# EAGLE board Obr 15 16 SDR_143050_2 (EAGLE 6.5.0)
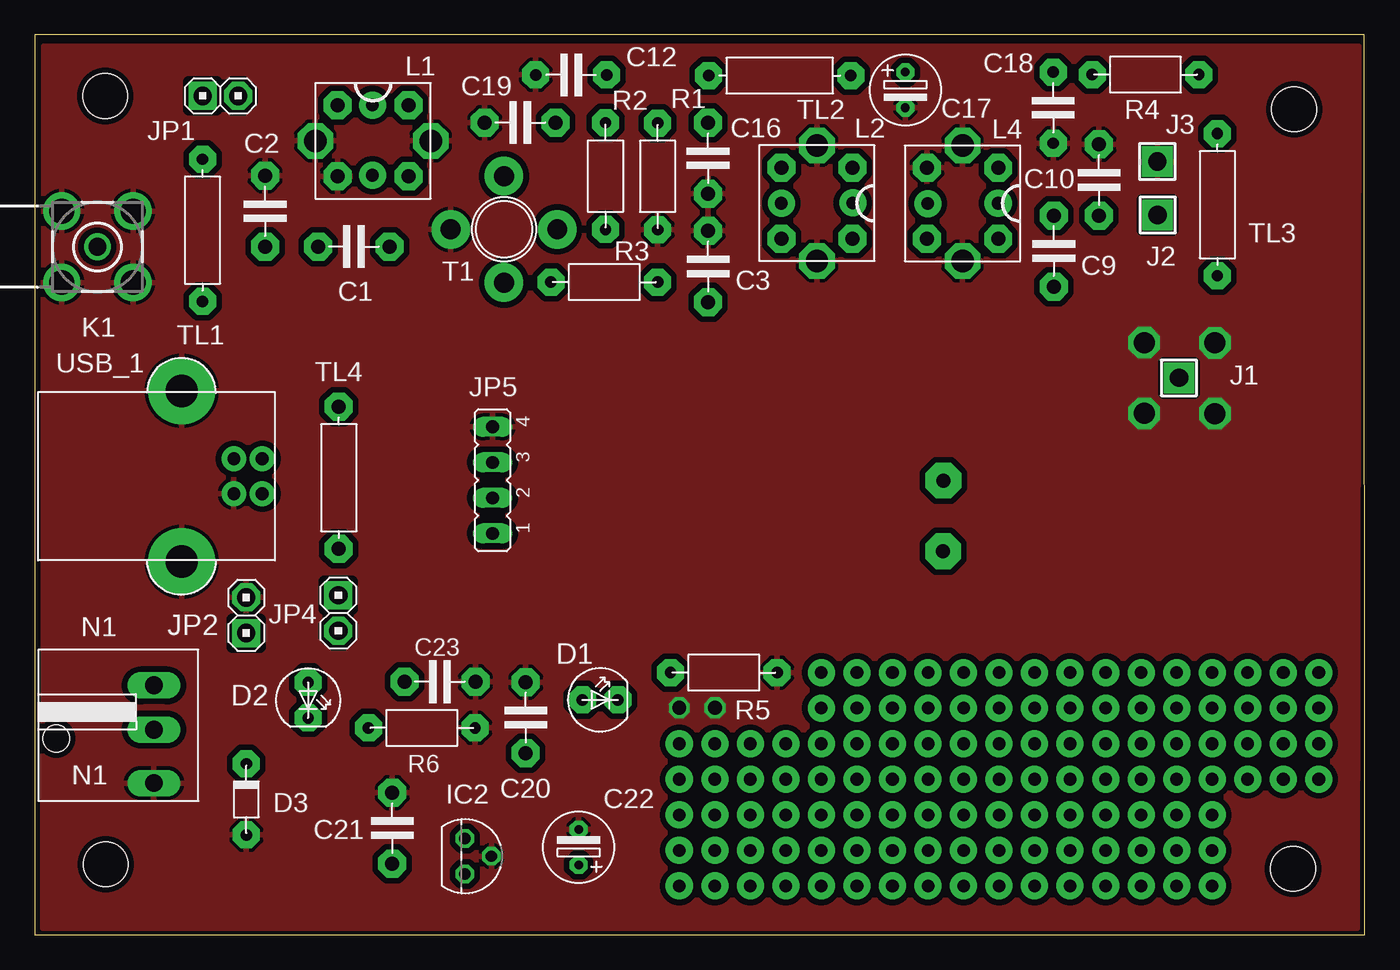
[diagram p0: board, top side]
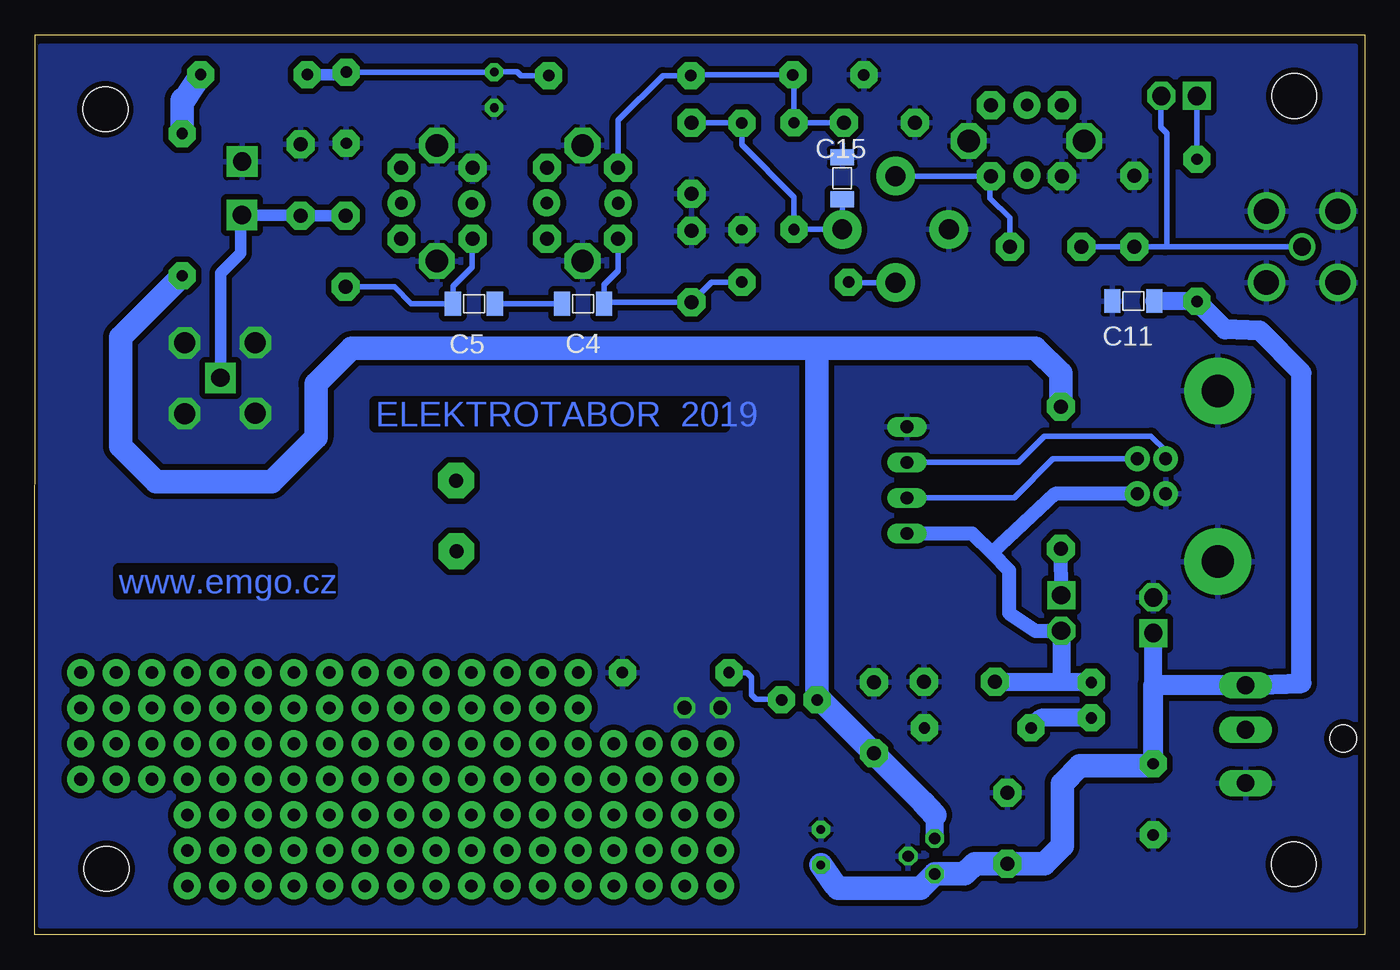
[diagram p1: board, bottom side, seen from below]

Size 95.05 x 64.29 mm. Coordinates in mm from the lower left corner, seen from the top.
Outline: 0,0 95.05,0 95.02,64.29 0,64.29 0,0
Copper layers (1*16): Top 0.035mm / dielectric 1.5mm / Bottom 0.035mm
Design rules "default *": minimum track width 10mil, minimum drill 24mil, track to track 8mil, track to pad 8mil, pad to pad 8mil, via to via 8mil, smd to smd 8mil, copper to edge 0mil, drill to drill 8mil, minimum pad ring 10mil, minimum via ring 8mil, stop-mask expansion 4mil, vias tented up to drill 0mil, thermal gap 10mil
Holes 3.2 mm at 5.05,5.02 90.01,59 89.94,4.72 5.02,59.94

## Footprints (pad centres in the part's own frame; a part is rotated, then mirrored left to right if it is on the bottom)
C-5 = drill 1 pad 2 octagon: 1 -2.54,0; 2 2.54,0
SMD-1206 = smd 1.15 x 1.7: 1 -1.5,0; 2 1.5,0
C-5@2 = drill 0.813 pad 1.93 octagon: 1 -2.54,0; 2 2.54,0
ES-2,5L = drill 0.61 pad 1.27 octagon: 1 0,0; 2 2.54,0
LED = drill 0.813 pad 1.93 octagon: A 0,0; K 2.54,0
D-5 = drill 0.813 pad 1.93 octagon: 1 -2.54,0; 2 2.54,0
TO92 = drill 0.813 octagon: 1 -1.27,0; 2 0,1.905; 3 1.27,0
PAD-01 = drill 1.3 pad 2.184 square: 1 0,0
PINH-2 = drill 1.3 pad 2 square: 1 0,0 | drill 1.3 pad 2 octagon: 2 2.54,0
JP4 = drill 0.914 long: 1 -3.81,0; 2 -1.27,0; 3 1.27,0; 4 3.81,0
BU-SMA-H = drill 1.27: 1 0,0 | drill 1.778: 2 -2.55,2.55; 3 2.55,2.55; 4 2.55,-2.55; 5 -2.55,-2.55
L-VF50 = drill 1 pad 2 octagon: 1 -2.54,-2.54; 2 2.54,-2.54; 3 2.54,2.54; 4 -2.54,2.54 | drill 1.6 pad 2.54 octagon: 5 -4.128,0; 6 4.128,0
NAPVIDL = drill 1.27 pad 1.905 long: 1 3.175,0; 2 -3.81,0; 3 0,0 | hole 1.93: -0.635,6.985
R-7,5 = drill 0.813 pad 1.93 octagon: 1 -3.81,0; 2 3.81,0
BF982 = drill 1.422 pad 2.75: 1 -3.81,0; 2 0,3.81; 3 3.81,0; 4 0,-3.81
L-10@2 = drill 0.813 pad 1.93 octagon: 1 -5.08,0; 2 5.08,0
L-10 = drill 1 pad 2 octagon: 1 -5.08,0; 2 5.08,0
USB1X90B = drill 0.92 pad 1.778: 1 -1.016,1.245; 2 -1.016,-1.245; 3 1.016,-1.245; 4 1.016,1.245 | drill 2.3 pad 4.778: P$3 4.75,-6.096; P$4 4.75,6.096

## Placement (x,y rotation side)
C1  5.6pF  [C-5]  22.8,49.17 0 top
C2  33pF  [C-5]  16.45,51.7 270 top
C3  8.2pF  [C-5]  48.12,47.75 270 top
C4  1pF  [SMD-1206]  55.87,45.09 0 bottom
C5  1pF  [SMD-1206]  63.67,45.09 0 bottom
C9  4.7pF  [C-5]  72.84,48.85 270 top
C10  33pF  [C-5]  76.07,53.93 270 top
C11  100nF  [SMD-1206]  16.53,45.28 180 bottom
C12  100nF  [C-5@2]  38.33,61.44 0 top
C15  1nF  [SMD-1206]  37.33,54.04 90 bottom
C16  100nF  [C-5]  48.12,55.48 270 top
C17  47uF  [ES-2,5L]  62.23,61.63 270 top
C18  100nF  [C-5@2]  72.79,59.1 90 top
C19  1nF  [C-5]  34.69,58.03 180 top
C20  100nF  [C-5]  35.08,15.51 270 top
C21  100nF  [C-5]  25.55,7.61 270 top
C22  47uF  [ES-2,5L]  38.86,4.98 90 top
C23  100nF  [C-5]  28.95,18.08 0 top
D1  RED/5mA  [LED]  39.14,16.78 0 top
D2  RED/5mA  [LED]  19.53,18.03 270 top
D3  protect  [D-5]  15.11,9.67 90 top
IC2  78L08Z  [TO92]  30.73,5.61 270 top
J1  [PAD-01]  81.78,39.8 90 top
J2  [PAD-01]  80.26,51.43 0 top
J3  [PAD-01]  80.23,55.25 0 top
JP1  [PINH-2]  11.98,59.94 0 top
JP2  UCC-GND  [PINH-2]  15.11,21.56 90 top
JP4  USB-GND  [PINH-2]  21.69,24.25 270 top
JP5  [JP4]  32.71,32.48 90 top
K1  [BU-SMA-H]  4.47,49.16 180 top
L1  [L-VF50]  24.17,56.73 0 top
L2  [L-VF50]  55.9,52.27 270 top
L4  [L-VF50]  66.31,52.26 270 top
N1  12V-DC  [NAPVIDL]  8.5,14.65 90 top
R1  100K  [R-7,5]  44.51,54.18 270 top
R2  100K  [R-7,5]  40.79,54.21 90 top
R3  47R  [R-7,5]  40.7,46.63 180 top
R4  2R2  [R-7,5]  79.39,61.46 180 top
R5  1K  [R-7,5]  49.24,18.73 180 top
R6  1K  [R-7,5]  27.66,14.78 180 top
T1  BF982A  [BF982]  33.53,50.4 0 top
TL1  10uH  [L-10@2]  11.98,50.34 270 top
TL2  TLUM  [L-10@2]  53.24,61.39 0 top
TL3  TLUM  [L-10@2]  84.53,52.17 270 top
TL4  10uH  [L-10]  21.72,32.65 270 top
USB_1  [USB1X90B]  15.24,32.76 180 top

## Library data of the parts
C1-C5 C9-C12 C15-C23 D1-D3 J1-J3 JP1 JP2 JP4 L1 L2 L4 N1 R1-R6 TL1-TL4 = M
IC2 = linear
JP5 = jumper
K1 = con-coax; OC_FARNELL: unknown; OC_NEWARK: unknown
T1 = transistor-fet
USB_1 = EMGO_BNC

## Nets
+12V: C11.1 C21.2 C22.1 D3.2 IC2.3 JP2.1 N1.1 TL1.2
+12V1: C23.1 D2.A JP4.2 JP5.1 USB_1.1
+12V2: C20.2 D1.A IC2.1 TL3.2 TL4.1
GND: C2.1 C3.1 C10.1 C11.2 C12.1 C15.2 C16.2 C17.2 C18.1 C19.2 C20.1 C21.1 C22.2 C23.2 D3.1 IC2.2 J3.1 JP2.2 JP5.4 K1.2 K1.3 K1.4 K1.5 L1.1 L1.5 L1.6 L2.5 L2.6 L4.1 L4.5 L4.6 N1.2 R1.2 R5.1 R6.1 T1.1 USB_1.4 USB_1.P$3 USB_1.P$4
N$1: R4.1 TL3.1
N$2: R3.2 T1.4
N$8: D2.K R6.2
N$10: JP5.2 USB_1.2
N$13: C17.1 C18.2 R4.2 TL2.2
N$14: JP5.3 USB_1.3
N$16: C4.1 C5.2
N$29: C5.1 C9.2 L4.2
N$30: C9.1 C10.2 J1.1 J2.1
N$34: JP1.1 TL1.1
N$36: C3.2 C4.2 L2.2 R3.1
N$38: C12.2 C19.1 L2.1 R2.2 TL2.1
N$44: C1.2 L1.2 T1.2
N$45: C1.1 C2.2 JP1.2 K1.1
N$50: C15.1 C16.1 R1.1 R2.1 T1.3
N$85: D1.K R5.2
N$146: JP4.1 TL4.2

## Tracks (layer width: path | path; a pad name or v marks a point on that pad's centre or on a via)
+12V
  Bottom 0.406: 15.03,45.26 C11.1
  Bottom 1.27: TL1.2 15.01,45.26 C11.1 | 15.11,17.82 JP2.1
  Bottom 1.422: TL1.2 9.98,43.25 7.49,43.17 4.52,40.15 4.52,17.98 N1.1 15.11,17.82 D3.2
  Bottom 1.676: C22.1 37.91,3.59 37.64,3.32 31.75,3.32 IC2.3 28.6,4.34 27.86,5.07 C21.2 22.88,5.07 21.61,6.34 21.61,10.79 20.34,12.06 15.26,12.06 D3.2
+12V1
  Bottom 1.016: JP5.1 28.06,28.67 26.65,27.31 | 26.65,27.31 25.42,26.03 25.42,22.98 23.52,21.71 JP4.2 | USB_1.1 22.13,31.5 26.65,27.31
  Bottom 1.27: C23.1 21.61,18.08 | 21.61,18.08 19.58,18.08 D2.A | JP4.2 21.69,18.15 21.61,18.08
+12V2
  Bottom 1.27: IC2.1 30.73,8.54
  Bottom 1.676: TL4.1 21.72,40.11 23.52,41.9 39.39,41.9 | 39.39,41.9 72.41,41.9 74.95,39.36 74.95,35.55 78.13,32.38 86.38,32.38 88.92,34.92 88.92,42.69 TL3.2 | 39.39,41.9 39.14,41.65 D1.A 38.89,16.78 C20.2 31.6,9.49 30.73,8.54
GND  (via drill 1 pad 1.02, 1.5)
  other vias: 46.06,16.21 48.62,16.21 79.29,42.31 84.35,42.28 84.35,37.23 79.29,37.26
  pour Bottom (isolate 0.406): 0.66,0.63 0.66,63.49 94.64,63.49 94.64,0.63
  pour Top (isolate 0.406): 0.63,63.49 94.64,63.49 94.53,0.48 0.55,0.48
N$1
  Bottom 1.676: TL3.1 84.53,59.63 84.48,59.68 84.34,59.68 R4.1
N$2
  Bottom 0.406: T1.4 36.84,46.59 R3.2
N$3  (via drill 0.9 pad 1.93)
  other vias: 46.06,13.65
N$8
  Bottom 1.27: D2.K 23.13,15.49 R6.2
N$9  (via drill 0.9 pad 1.93)
  other vias: 48.6,13.65
N$10
  Bottom 0.406: USB_1.2 22.27,34 25.04,31.24 JP5.2
N$11  (via drill 0.9 pad 1.93)
  other vias: 51.14,13.65
N$12  (via drill 0.9 pad 1.93)
  other vias: 53.68,13.65
N$13
  Bottom 0.406: C18.2 C17.1 62.19,61.66 60.57,61.66 60.3,61.39 TL2.2
  Bottom 0.813: R4.2 72.96,61.46 C18.2
N$14
  Bottom 0.406: JP5.3 24.73,33.78 22.88,35.63 15.26,35.63 14.22,34.59 USB_1.3
N$15  (via drill 0.9 pad 1.93)
  other vias: 46.06,11.11
N$16
  Bottom 0.406: C4.1 C5.2
N$17  (via drill 0.9 pad 1.93)
  other vias: 48.6,11.11
N$19  (via drill 0.9 pad 1.93)
  other vias: 51.14,11.11
N$20  (via drill 0.9 pad 1.93)
  other vias: 53.68,11.11
N$21  (via drill 0.9 pad 1.93)
  other vias: 46.06,8.57
N$22  (via drill 0.9 pad 1.93)
  other vias: 48.6,8.57
N$23  (via drill 0.9 pad 1.93)
  other vias: 51.14,8.57
N$24  (via drill 0.9 pad 1.93)
  other vias: 53.68,8.57
N$25  (via drill 0.9 pad 1.93)
  other vias: 48.6,6.03
N$26  (via drill 0.9 pad 1.93)
  other vias: 53.68,6.03
N$27  (via drill 0.9 pad 1.93)
  other vias: 51.14,6.03
N$28  (via drill 0.9 pad 1.93)
  other vias: 46.06,6.03
N$29
  Bottom 0.406: L4.2 63.8,49.69 63.8,47.69 65.17,46.32 C5.1 65.19,45.1 68.14,45.1 69.35,46.31 C9.2
N$30
  Bottom 0.813: C9.1 C10.2 76.11,51.43 J2.1 80.34,51.35 80.34,48.71 81.78,47.26 J1.1
N$31  (via drill 0.9 pad 1.93)
  other vias: 46.06,3.49
N$32  (via drill 0.9 pad 1.93)
  other vias: 48.6,3.49
N$33  (via drill 0.9 pad 1.93)
  other vias: 51.14,3.49
N$34
  Bottom 0.406: TL1.1 JP1.1
N$35  (via drill 0.9 pad 1.93)
  other vias: 53.68,3.49
N$36
  Bottom 0.406: L2.2 53.36,47.44 54.37,46.43 C4.2 54.25,45.21 C3.2 46.7,46.63 R3.1
N$37  (via drill 0.9 pad 1.93)
  other vias: 56.22,3.49
N$38
  Bottom 0.406: C19.1 40.77,58.03 R2.2 40.79,61.35 C12.2 48.12,61.44 TL2.1 50.16,61.39 53.36,58.18 L2.1
N$39  (via drill 0.9 pad 1.93)
  other vias: 56.22,6.03
N$40  (via drill 0.9 pad 1.93)
  other vias: 56.22,8.57
N$41  (via drill 0.9 pad 1.93)
  other vias: 56.22,11.11
N$42  (via drill 0.9 pad 1.93)
  other vias: 56.22,13.65
N$43  (via drill 0.9 pad 1.93)
  other vias: 56.22,16.19
N$44
  Bottom 0.406: T1.2 33.53,54.19 L1.2 26.77,54.13 26.77,52.62 25.37,51.23 25.37,49.17 C1.2
N$45
  Bottom 0.406: K1.1 14.27,49.16 | 14.27,49.16 C2.2 C1.1 | 14.27,49.16 14.14,49.28 14.14,57.27 14.57,57.7 14.57,59.89 JP1.2
N$46  (via drill 0.9 pad 1.93)
  other vias: 56.22,18.73
N$47  (via drill 0.9 pad 1.93)
  other vias: 58.76,6.03
N$48  (via drill 0.9 pad 1.93)
  other vias: 58.76,16.19
N$49  (via drill 0.9 pad 1.93)
  other vias: 58.76,13.65
N$50
  Bottom 0.406: 37.33,50.41 T1.3 | T1.3 R2.1 40.79,52.7 44.52,56.43 R1.1 44.54,58.02 C16.1 | T1.3 C15.1
N$51  (via drill 0.9 pad 1.93)
  other vias: 58.76,11.11
N$52  (via drill 0.9 pad 1.93)
  other vias: 58.76,8.57
N$53  (via drill 0.9 pad 1.93)
  other vias: 58.76,3.49
N$54  (via drill 0.9 pad 1.93)
  other vias: 58.76,18.73
N$55  (via drill 0.9 pad 1.93)
  other vias: 61.3,6.03
N$56  (via drill 0.9 pad 1.93)
  other vias: 61.3,16.19
N$57  (via drill 0.9 pad 1.93)
  other vias: 61.3,13.65
N$58  (via drill 0.9 pad 1.93)
  other vias: 61.3,11.11
N$59  (via drill 0.9 pad 1.93)
  other vias: 61.3,8.57
N$60  (via drill 0.9 pad 1.93)
  other vias: 84.16,6.03
N$61  (via drill 0.9 pad 1.93)
  other vias: 61.3,3.49
N$62  (via drill 0.9 pad 1.93)
  other vias: 63.84,3.49
N$63  (via drill 0.9 pad 1.93)
  other vias: 63.84,6.03
N$64  (via drill 0.9 pad 1.93)
  other vias: 63.84,8.57
N$65  (via drill 0.9 pad 1.93)
  other vias: 63.84,11.11
N$66  (via drill 0.9 pad 1.93)
  other vias: 63.84,13.65
N$67  (via drill 0.9 pad 1.93)
  other vias: 63.84,16.19
N$68  (via drill 0.9 pad 1.93)
  other vias: 61.3,18.73
N$69  (via drill 0.9 pad 1.93)
  other vias: 63.84,18.73
N$70  (via drill 0.9 pad 1.93)
  other vias: 66.38,6.03
N$71  (via drill 0.9 pad 1.93)
  other vias: 66.38,18.73
N$72  (via drill 0.9 pad 1.93)
  other vias: 66.38,16.19
N$73  (via drill 0.9 pad 1.93)
  other vias: 66.38,13.65
N$74  (via drill 0.9 pad 1.93)
  other vias: 66.38,11.11
N$75  (via drill 0.9 pad 1.93)
  other vias: 66.38,8.57
N$76  (via drill 0.9 pad 1.93)
  other vias: 24.12,54.27
N$77  (via drill 0.9 pad 1.93)
  other vias: 24.12,59.28
N$78  (via drill 0.9 pad 1.93)
  other vias: 53.36,52.27
N$79  (via drill 0.9 pad 1.93)
  other vias: 58.47,52.29
N$80  (via drill 0.9 pad 1.93)
  other vias: 63.83,52.24
N$81  (via drill 0.9 pad 1.93)
  other vias: 68.85,52.27
N$82  (via drill 1 pad 2.54)
  other vias: 64.94,32.45
N$83  (via drill 1 pad 2.54)
  other vias: 64.92,27.4
N$84  (via drill 0.9 pad 1.93)
  other vias: 66.38,3.49
N$85
  Bottom 0.406: R5.2 44.16,18.73 43.84,18.41 43.84,17.14 43.52,16.82 41.71,16.82 D1.K
N$86  (via drill 0.9 pad 1.93)
  other vias: 68.92,3.49
N$87  (via drill 0.9 pad 1.93)
  other vias: 68.92,6.03
N$88  (via drill 0.9 pad 1.93)
  other vias: 68.92,8.57
N$89  (via drill 0.9 pad 1.93)
  other vias: 68.92,11.11
N$90  (via drill 0.9 pad 1.93)
  other vias: 68.92,13.65
N$91  (via drill 0.9 pad 1.93)
  other vias: 68.92,16.19
N$92  (via drill 0.9 pad 1.93)
  other vias: 68.92,18.73
N$93  (via drill 0.9 pad 1.93)
  other vias: 71.46,6.03
N$94  (via drill 0.9 pad 1.93)
  other vias: 71.46,18.73
N$95  (via drill 0.9 pad 1.93)
  other vias: 71.46,16.19
N$96  (via drill 0.9 pad 1.93)
  other vias: 71.46,13.65
N$97  (via drill 0.9 pad 1.93)
  other vias: 71.46,11.11
N$98  (via drill 0.9 pad 1.93)
  other vias: 71.46,8.57
N$99  (via drill 0.9 pad 1.93)
  other vias: 71.46,3.49
N$100  (via drill 0.9 pad 1.93)
  other vias: 74,3.49
N$101  (via drill 0.9 pad 1.93)
  other vias: 74,6.03
N$102  (via drill 0.9 pad 1.93)
  other vias: 74,8.57
N$103  (via drill 0.9 pad 1.93)
  other vias: 74,11.11
N$104  (via drill 0.9 pad 1.93)
  other vias: 74,13.65
N$105  (via drill 0.9 pad 1.93)
  other vias: 74,16.19
N$106  (via drill 0.9 pad 1.93)
  other vias: 74,18.73
N$107  (via drill 0.9 pad 1.93)
  other vias: 76.54,6.03
N$108  (via drill 0.9 pad 1.93)
  other vias: 76.54,16.19
N$109  (via drill 0.9 pad 1.93)
  other vias: 76.54,13.65
N$110  (via drill 0.9 pad 1.93)
  other vias: 76.54,11.11
N$111  (via drill 0.9 pad 1.93)
  other vias: 76.54,8.57
N$112  (via drill 0.9 pad 1.93)
  other vias: 76.54,3.49
N$113  (via drill 0.9 pad 1.93)
  other vias: 79.08,3.49
N$114  (via drill 0.9 pad 1.93)
  other vias: 79.08,6.03
N$115  (via drill 0.9 pad 1.93)
  other vias: 79.08,8.57
N$116  (via drill 0.9 pad 1.93)
  other vias: 79.08,11.11
N$117  (via drill 0.9 pad 1.93)
  other vias: 79.08,13.65
N$118  (via drill 0.9 pad 1.93)
  other vias: 79.08,16.19
N$119  (via drill 0.9 pad 1.93)
  other vias: 76.54,18.73
N$120  (via drill 0.9 pad 1.93)
  other vias: 79.08,18.73
N$121  (via drill 0.9 pad 1.93)
  other vias: 81.62,18.73
N$122  (via drill 0.9 pad 1.93)
  other vias: 84.16,18.73
N$123  (via drill 0.9 pad 1.93)
  other vias: 86.7,18.73
N$124  (via drill 0.9 pad 1.93)
  other vias: 89.24,18.73
N$125  (via drill 0.9 pad 1.93)
  other vias: 91.78,18.73
N$126  (via drill 0.9 pad 1.93)
  other vias: 86.7,16.19
N$127  (via drill 0.9 pad 1.93)
  other vias: 91.78,16.19
N$128  (via drill 0.9 pad 1.93)
  other vias: 89.24,16.19
N$129  (via drill 0.9 pad 1.93)
  other vias: 81.62,16.19
N$130  (via drill 0.9 pad 1.93)
  other vias: 84.16,16.19
N$131  (via drill 0.9 pad 1.93)
  other vias: 84.16,13.65
N$132  (via drill 0.9 pad 1.93)
  other vias: 81.62,13.65
N$133  (via drill 0.9 pad 1.93)
  other vias: 86.7,13.65
N$134  (via drill 0.9 pad 1.93)
  other vias: 89.24,13.65
N$135  (via drill 0.9 pad 1.93)
  other vias: 91.78,13.65
N$136  (via drill 0.9 pad 1.93)
  other vias: 91.78,11.11
N$137  (via drill 0.9 pad 1.93)
  other vias: 89.24,11.11
N$138  (via drill 0.9 pad 1.93)
  other vias: 86.7,11.11
N$139  (via drill 0.9 pad 1.93)
  other vias: 81.62,11.11
N$140  (via drill 0.9 pad 1.93)
  other vias: 84.16,11.11
N$141  (via drill 0.9 pad 1.93)
  other vias: 84.16,8.57
N$142  (via drill 0.9 pad 1.93)
  other vias: 81.62,8.57
N$143  (via drill 0.9 pad 1.93)
  other vias: 84.16,3.49
N$144  (via drill 0.9 pad 1.93)
  other vias: 81.62,6.03
N$145  (via drill 0.9 pad 1.93)
  other vias: 81.62,3.49
N$146
  Bottom 1.016: JP4.1 TL4.2

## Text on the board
Bottom: ELEKTROTABOR 2019 | www.emgo.cz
